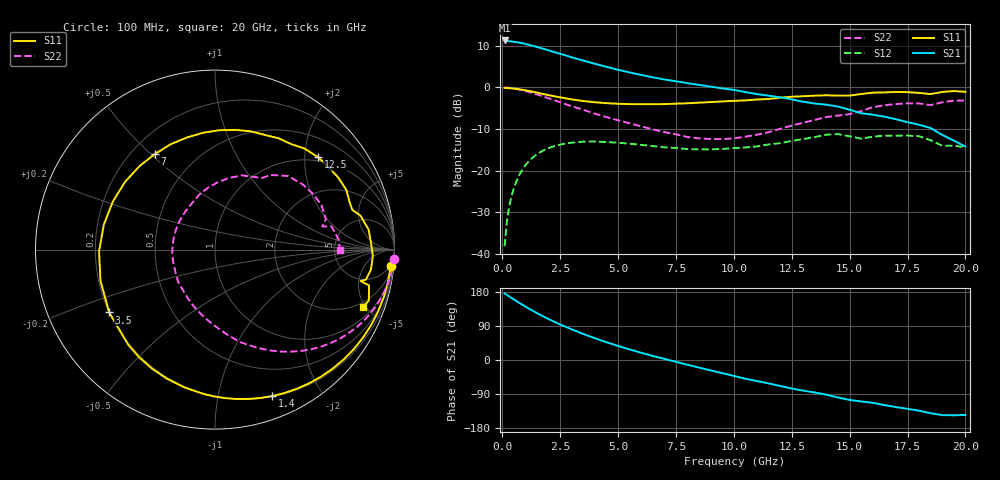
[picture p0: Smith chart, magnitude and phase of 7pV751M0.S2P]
! Infineon Technologies  Discrete & RF Semiconductors
! bfp620
! VCE = 0.75 V,  IC =  1.0 mA
! Common Emitter S-Parameters:  Sep 2002
# GHz  S  MA  R  50
!  f  S11  S21  S12  S22
! GHz  MAG  ANG  MAG  ANG  MAG  ANG  MAG  ANG
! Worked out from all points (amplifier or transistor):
!   59 points, 100 MHz to 20 GHz, reference 50 ohm
!   highest |S21| = 11.3 dB at 100 MHz (marker M1)
!   |S21| within 3 dB of that: start of sweep to 2.365 GHz
!   unconditionally stable (mu >= 1): 6.408 GHz to 15.94 GHz; 17.44 GHz to end of sweep
!   at 1 GHz: K = 0.12, MSG = 14.6 dB, |S12| = -18.7 dB
!   at 5.5 GHz: K = 0.82, MSG = 8.6 dB, |S12| = -13.6 dB
!   at 20 GHz: K = 1.84, MAG = -5.2 dB, |S12| = -14.4 dB
!   S11 on the Smith chart (normalised r, x): 100 MHz: 4, -21; 1.4 GHz: 0.21, -1.44; 3.5 GHz: 0.20, -0.26; 7 GHz: 0.29, +0.52; 12.5 GHz: 0.91, +2.31; 20 GHz: 1.65, -4.83
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0.1  0.9841 -5.4  3.667 175.5  0.0123 85.6  0.9992 -3.1
0.2  0.9808 -10.4  3.621 171.6  0.0247 83.5  0.9941 -6.2
0.3  0.977 -15.5  3.588 167.6  0.0371 80.7  0.9871 -9.2
0.5  0.9666 -25.6  3.532 159.7  0.0614 74.2  0.9686 -14.9
0.9  0.9326 -45.4  3.376 144.6  0.1057 61.1  0.9179 -25.7
1.4  0.8759 -68.7  3.114 127.0  0.1498 46.2  0.8384 -37.6
1.8  0.8291 -86.2  2.895 114.1  0.1756 35.8  0.7717 -46.0
2.2  0.7863 -102.6  2.679 102.2  0.1945 26.6  0.7084 -53.4
2.8  0.7332 -125.4  2.396 86.0  0.2123 14.5  0.6189 -63.8
3.5  0.6855 -149.3  2.101 68.7  0.2226 2.1  0.5357 -74.6
4  0.6617 -164.7  1.92 57.4  0.223 -5.7  0.4821 -81.3
5  0.6349 167.3  1.629 37.1  0.2158 -17.5  0.4021 -94.5
6  0.6273 143.1  1.412 19.1  0.2036 -26.5  0.34 -109.9
7  0.6292 122.2  1.244 3.1  0.1902 -32.1  0.2897 -127.6
8.5  0.6546 95.7  1.072 -20.0  0.1796 -36.4  0.2434 -163.4
10.5  0.6968 66.3  0.878 -49.4  0.1894 -40.6  0.2551 140.0
12.5  0.7715 41.9  0.717 -75.2  0.2268 -47.7  0.3471 96.4
13.5  0.7953 30.3  0.639 -85.7  0.2527 -55.7  0.4064 79.0
16  0.8632 7.4  0.469 -112.9  0.2552 -79.1  0.5788 45.1
17  0.8801 -2.4  0.414 -124.2  0.2627 -90.5  0.6296 29.2
18.5  0.8301 -12.2  0.324 -140.5  0.231 -113.1  0.6115 12.2
20  0.8846 -21.1  0.194 -145.0  0.1905 -116.8  0.6957 -0.3
